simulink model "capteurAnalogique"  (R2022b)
settings: Solver=VariableStepAuto  StartTime=0.0  StopTime=10.0  RelTol=1e-3  EnableMultiTasking=on
libraries: simulink x1

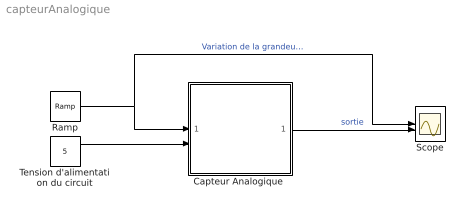
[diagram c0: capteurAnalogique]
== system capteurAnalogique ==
  "Capteur Analogique " : Subsystem  mask{gain=360}
      mask prompts: gain "Coefficient directeur"
  Ramp : simulink/Sources/Ramp  slope=36  start=0  InitialOutput=0
  Scope : Scope  NumInputPorts=2
  Tension d'alimentation du circuit : Constant  Value=5
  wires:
  Ramp/1 -> "Capteur Analogique "/1(thêta degré), Scope/1  "Variation de la grandeur d'entrée"
  "Capteur Analogique "/1(valeur capteur) -> Scope/2  "sortie"
  Tension d'alimentation du circuit/1 -> "Capteur Analogique "/2(tensionAlim)

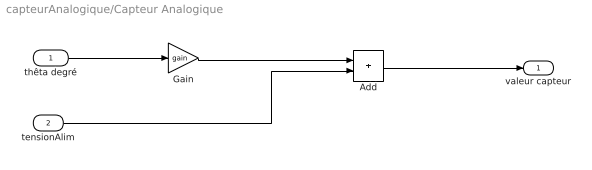
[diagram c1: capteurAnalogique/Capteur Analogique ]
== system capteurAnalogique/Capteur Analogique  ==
  thêta degré : Inport
  tensionAlim : Inport  Port=2
  Add : Sum
  Gain : Gain  Gain=gain
  valeur capteur : Outport  VectorParamsAs1DForOutWhenUnconnected=off
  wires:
  thêta degré/1 -> Gain/1
  Gain/1 -> Add/1
  Add/1 -> valeur capteur/1
  tensionAlim/1 -> Add/2
